| / 7\'7   Xilinx XC9500 I/O Buffer IBIS File
| \ \   Xilinx Inc.
| / /   2100 Logic Drive
| \_\/.\   San Jose,   CA 95124
[IBIS ver]   2.1
[File name]   xc9500.ibs
[File Rev]   1.2
[Date]   June 15, 1999
[Source]   Spice netlist
[Notes]   - max/min process data is not included in this ibis model
   - Control flag setting:
   SLW=0 - fast slew rate
   SLW=1 - slow slew rate
   VIO=0 - 3.3V Vddio
   VIO=1 - 5.0V Vddio
   - Created by Joey Jia x4437
[Disclaimer] The data in this model is derived from SPICE simulations
   using modeling information extracted from the target pro-
   cess. While a great deal of care has been take to provide
   information that is accurate, this model is considered
   preliminary as it has not been verified by actual silicon
   measurement. Treat the data in this model as preliminary
   until actual silicon verification is performed.
[Copyright]   Xilinx Inc.
|   Component XC9536_PLCC44[SLW=0;VIO=0]
[Component]   XC9536_PLCC44[SLW=0;VIO=0]
[Manufacturer]   Xilinx Inc.
[Package]
| variable   typ   min   max
R_pkg   67.500m   66.000m   69.000m
L_pkg   3.910nH   3.550nH   4.260nH
C_pkg   0.895pF   0.790pF   1.000pF
[Pin]  signal_name   model_name   R_pin   L_pin   C_pin
io   iob   IO_00   NA   NA   NA
|   Component XC9536_PLCC44[SLW=1;VIO=0]
[Component]   XC9536_PLCC44[SLW=1;VIO=0]
[Manufacturer]   Xilinx Inc.
[Package]
| variable   typ   min   max
R_pkg   67.500m   66.000m   69.000m
L_pkg   3.910nH   3.550nH   4.260nH
C_pkg   0.895pF   0.790pF   1.000pF
[Pin]  signal_name   model_name   R_pin   L_pin   C_pin
io   iob   IO_10   NA   NA   NA
|   Component XC9536_PLCC44[SLW=0;VIO=1]
[Component]   XC9536_PLCC44[SLW=0;VIO=1]
[Manufacturer]   Xilinx Inc.
[Package]
| variable   typ   min   max
R_pkg   67.500m   66.000m   69.000m
L_pkg   3.910nH   3.550nH   4.260nH
C_pkg   0.895pF   0.790pF   1.000pF
[Pin]  signal_name   model_name   R_pin   L_pin   C_pin
io   iob   IO_01   NA   NA   NA
|   Component XC9536_PLCC44[SLW=1;VIO=1]
[Component]   XC9536_PLCC44[SLW=1;VIO=1]
[Manufacturer]   Xilinx Inc.
[Package]
| variable   typ   min   max
R_pkg   67.500m   66.000m   69.000m
L_pkg   3.910nH   3.550nH   4.260nH
C_pkg   0.895pF   0.790pF   1.000pF
[Pin]  signal_name   model_name   R_pin   L_pin   C_pin
io   iob   IO_11   NA   NA   NA
|   Component XC9536_VQ44[SLW=0;VIO=0]
[Component]   XC9536_VQ44[SLW=0;VIO=0]
[Manufacturer]   Xilinx Inc.
[Package]
| variable   typ   min   max
R_pkg   57.000m   54.000m   60.000m
L_pkg   2.270nH   2.100nH   2.430nH
C_pkg   0.275pF   0.260pF   0.290pF
[Pin]  signal_name   model_name   R_pin   L_pin   C_pin
io   iob   IO_00   NA   NA   NA
| End [Component] XC9536_VQ44[SLW=0;VIO=0]
|   Component XC9536_VQ44[SLW=0;VIO=1]
[Component]   XC9536_VQ44[SLW=0;VIO=1]
[Manufacturer]   Xilinx Inc.
[Package]
| variable   typ   min   max
R_pkg   57.000m   54.000m   60.000m
L_pkg   2.270nH   2.100nH   2.430nH
C_pkg   0.275pF   0.260pF   0.290pF
[Pin]  signal_name   model_name   R_pin   L_pin   C_pin
io   iob   IO_01   NA   NA   NA
| End [Component] XC9536_VQ44[SLW=0;VIO=1]
|   Component XC9536_VQ44[SLW=1;VIO=0]
[Component]   XC9536_VQ44[SLW=1;VIO=0]
[Manufacturer]   Xilinx Inc.
[Package]
| variable   typ   min   max
R_pkg   57.000m   54.000m   60.000m
L_pkg   2.270nH   2.100nH   2.430nH
C_pkg   0.275pF   0.260pF   0.290pF
[Pin]  signal_name   model_name   R_pin   L_pin   C_pin
io   iob   IO_10   NA   NA   NA
| End [Component] XC9536_VQ44[SLW=1;VIO=0]
|   Component XC9536_VQ44[SLW=1;VIO=1]
[Component]   XC9536_VQ44[SLW=1;VIO=1]
[Manufacturer]   Xilinx Inc.
[Package]
| variable   typ   min   max
R_pkg   57.000m   54.000m   60.000m
L_pkg   2.270nH   2.100nH   2.430nH
C_pkg   0.275pF   0.260pF   0.290pF
[Pin]  signal_name   model_name   R_pin   L_pin   C_pin
io   iob   IO_11   NA   NA   NA
| End [Component] XC9536_VQ44[SLW=1;VIO=1]
|   Component XC9572_PLCC44[SLW=0;VIO=0]
[Component]   XC9572_PLCC44[SLW=0;VIO=0]
[Manufacturer]   Xilinx Inc.
[Package]
| variable   typ   min   max
R_pkg   67.500m   66.000m   69.000m
L_pkg   3.910nH   3.550nH   4.260nH
C_pkg   0.895pF   0.790pF   1.000pF
[Pin]  signal_name   model_name   R_pin   L_pin   C_pin
io   iob   IO_00   NA   NA   NA
| End [Component] XC9572_PLCC44[SLW=0;VIO=0]
|   Component XC9572_PLCC44[SLW=0;VIO=1]
[Component]   XC9572_PLCC44[SLW=0;VIO=1]
[Manufacturer]   Xilinx Inc.
[Package]
| variable   typ   min   max
R_pkg   67.500m   66.000m   69.000m
L_pkg   3.910nH   3.550nH   4.260nH
C_pkg   0.895pF   0.790pF   1.000pF
[Pin]  signal_name   model_name   R_pin   L_pin   C_pin
io   iob   IO_01   NA   NA   NA
| End [Component] XC9572_PLCC44[SLW=0;VIO=1]
|   Component XC9572_PLCC44[SLW=1;VIO=0]
[Component]   XC9572_PLCC44[SLW=1;VIO=0]
[Manufacturer]   Xilinx Inc.
[Package]
| variable   typ   min   max
R_pkg   67.500m   66.000m   69.000m
L_pkg   3.910nH   3.550nH   4.260nH
C_pkg   0.895pF   0.790pF   1.000pF
[Pin]  signal_name   model_name   R_pin   L_pin   C_pin
io   iob   IO_10   NA   NA   NA
| End [Component] XC9572_PLCC44[SLW=1;VIO=0]
|   Component XC9572_PLCC44[SLW=1;VIO=1]
[Component]   XC9572_PLCC44[SLW=1;VIO=1]
[Manufacturer]   Xilinx Inc.
[Package]
| variable   typ   min   max
R_pkg   67.500m   66.000m   69.000m
L_pkg   3.910nH   3.550nH   4.260nH
C_pkg   0.895pF   0.790pF   1.000pF
[Pin]  signal_name   model_name   R_pin   L_pin   C_pin
io   iob   IO_11   NA   NA   NA
| End [Component] XC9572_PLCC44[SLW=1;VIO=1]
|   Component XC9572_PLCC84[SLW=0;VIO=0]
[Component]   XC9572_PLCC84[SLW=0;VIO=0]
[Manufacturer]   Xilinx Inc.
[Package]
| variable   typ   min   max
R_pkg   0.104   97.000m   0.111
L_pkg   11.600nH   10.200nH   13.000nH
C_pkg   1.700pF   1.600pF   1.800pF
[Pin]  signal_name   model_name   R_pin   L_pin   C_pin
io   iob   IO_00   NA   NA   NA
| End [Component] XC9572_PLCC84[SLW=0;VIO=0]
|   Component XC9572_PLCC84[SLW=0;VIO=1]
[Component]   XC9572_PLCC84[SLW=0;VIO=1]
[Manufacturer]   Xilinx Inc.
[Package]
| variable   typ   min   max
R_pkg   0.104   97.000m   0.111
L_pkg   11.600nH   10.200nH   13.000nH
C_pkg   1.700pF   1.600pF   1.800pF
[Pin]  signal_name   model_name   R_pin   L_pin   C_pin
io   iob   IO_01   NA   NA   NA
| End [Component] XC9572_PLCC84[SLW=0;VIO=1]
|   Component XC9572_PLCC84[SLW=1;VIO=0]
[Component]   XC9572_PLCC84[SLW=1;VIO=0]
[Manufacturer]   Xilinx Inc.
[Package]
| variable   typ   min   max
R_pkg   0.104   97.000m   0.111
L_pkg   11.600nH   10.200nH   13.000nH
C_pkg   1.700pF   1.600pF   1.800pF
[Pin]  signal_name   model_name   R_pin   L_pin   C_pin
io   iob   IO_10   NA   NA   NA
| End [Component] XC9572_PLCC84[SLW=1;VIO=0]
|   Component XC9572_PLCC84[SLW=1;VIO=1]
[Component]   XC9572_PLCC84[SLW=1;VIO=1]
[Manufacturer]   Xilinx Inc.
[Package]
| variable   typ   min   max
R_pkg   0.104   97.000m   0.111
L_pkg   11.600nH   10.200nH   13.000nH
C_pkg   1.700pF   1.600pF   1.800pF
[Pin]  signal_name   model_name   R_pin   L_pin   C_pin
io   iob   IO_11   NA   NA   NA
| End [Component] XC9572_PLCC84[SLW=1;VIO=1]
|   Component XC9572_PQ100[SLW=0;VIO=0]
[Component]   XC9572_PQ100[SLW=0;VIO=0]
[Manufacturer]   Xilinx Inc.
[Package]
| variable   typ   min   max
R_pkg   88.000m   78.000m   98.000m
L_pkg   6.100nH   4.100nH   8.100nH
C_pkg   0.900pF   0.700pF   1.100pF
[Pin]  signal_name   model_name   R_pin   L_pin   C_pin
io   iob   IO_00   NA   NA   NA
| End [Component] XC9572_PQ100[SLW=0;VIO=0]
|   Component XC9572_PQ100[SLW=0;VIO=1]
[Component]   XC9572_PQ100[SLW=0;VIO=1]
[Manufacturer]   Xilinx Inc.
[Package]
| variable   typ   min   max
R_pkg   88.000m   78.000m   98.000m
L_pkg   6.100nH   4.100nH   8.100nH
C_pkg   0.900pF   0.700pF   1.100pF
[Pin]  signal_name   model_name   R_pin   L_pin   C_pin
io   iob   IO_01   NA   NA   NA
| End [Component] XC9572_PQ100[SLW=0;VIO=1]
|   Component XC9572_PQ100[SLW=1;VIO=0]
[Component]   XC9572_PQ100[SLW=1;VIO=0]
[Manufacturer]   Xilinx Inc.
[Package]
| variable   typ   min   max
R_pkg   88.000m   78.000m   98.000m
L_pkg   6.100nH   4.100nH   8.100nH
C_pkg   0.900pF   0.700pF   1.100pF
[Pin]  signal_name   model_name   R_pin   L_pin   C_pin
io   iob   IO_10   NA   NA   NA
| End [Component] XC9572_PQ100[SLW=1;VIO=0]
|   Component XC9572_PQ100[SLW=1;VIO=1]
[Component]   XC9572_PQ100[SLW=1;VIO=1]
[Manufacturer]   Xilinx Inc.
[Package]
| variable   typ   min   max
R_pkg   88.000m   78.000m   98.000m
L_pkg   6.100nH   4.100nH   8.100nH
C_pkg   0.900pF   0.700pF   1.100pF
[Pin]  signal_name   model_name   R_pin   L_pin   C_pin
io   iob   IO_11   NA   NA   NA
| End [Component] XC9572_PQ100[SLW=1;VIO=1]
|   Component XC9572_TQ100[SLW=0;VIO=0]
[Component]   XC9572_TQ100[SLW=0;VIO=0]
[Manufacturer]   Xilinx Inc.
[Package]
| variable   typ   min   max
R_pkg   84.500m   79.000m   90.000m
L_pkg   4.370nH   3.820nH   4.920nH
C_pkg   0.610pF   0.570pF   0.650pF
[Pin]  signal_name   model_name   R_pin   L_pin   C_pin
io   iob   IO_00   NA   NA   NA
| End [Component] XC9572_TQ100[SLW=0;VIO=0]
|   Component XC9572_TQ100[SLW=0;VIO=1]
[Component]   XC9572_TQ100[SLW=0;VIO=1]
[Manufacturer]   Xilinx Inc.
[Package]
| variable   typ   min   max
R_pkg   84.500m   79.000m   90.000m
L_pkg   4.370nH   3.820nH   4.920nH
C_pkg   0.610pF   0.570pF   0.650pF
[Pin]  signal_name   model_name   R_pin   L_pin   C_pin
io   iob   IO_01   NA   NA   NA
| End [Component] XC9572_TQ100[SLW=0;VIO=1]
|   Component XC9572_TQ100[SLW=1;VIO=0]
[Component]   XC9572_TQ100[SLW=1;VIO=0]
[Manufacturer]   Xilinx Inc.
[Package]
| variable   typ   min   max
R_pkg   84.500m   79.000m   90.000m
L_pkg   4.370nH   3.820nH   4.920nH
C_pkg   0.610pF   0.570pF   0.650pF
[Pin]  signal_name   model_name   R_pin   L_pin   C_pin
io   iob   IO_10   NA   NA   NA
| End [Component] XC9572_TQ100[SLW=1;VIO=0]
|   Component XC9572_TQ100[SLW=1;VIO=1]
[Component]   XC9572_TQ100[SLW=1;VIO=1]
[Manufacturer]   Xilinx Inc.
[Package]
| variable   typ   min   max
R_pkg   84.500m   79.000m   90.000m
L_pkg   4.370nH   3.820nH   4.920nH
C_pkg   0.610pF   0.570pF   0.650pF
[Pin]  signal_name   model_name   R_pin   L_pin   C_pin
io   iob   IO_11   NA   NA   NA
| End [Component] XC9572_TQ100[SLW=1;VIO=1]
|   Component XC95108_PLCC84[SLW=0;VIO=0]
[Component]   XC95108_PLCC84[SLW=0;VIO=0]
[Manufacturer]   Xilinx Inc.
[Package]
| variable   typ   min   max
R_pkg   0.104   97.000m   0.111
L_pkg   11.600nH   10.200nH   13.000nH
C_pkg   1.700pF   1.600pF   1.800pF
[Pin]  signal_name   model_name   R_pin   L_pin   C_pin
io   iob   IO_00   NA   NA   NA
| End [Component] XC95108_PLCC84[SLW=0;VIO=0]
|   Component XC95108_PLCC84[SLW=0;VIO=1]
[Component]   XC95108_PLCC84[SLW=0;VIO=1]
[Manufacturer]   Xilinx Inc.
[Package]
| variable   typ   min   max
R_pkg   0.104   97.000m   0.111
L_pkg   11.600nH   10.200nH   13.000nH
C_pkg   1.700pF   1.600pF   1.800pF
[Pin]  signal_name   model_name   R_pin   L_pin   C_pin
io   iob   IO_01   NA   NA   NA
| End [Component] XC95108_PLCC84[SLW=0;VIO=1]
|   Component XC95108_PLCC84[SLW=1;VIO=0]
[Component]   XC95108_PLCC84[SLW=1;VIO=0]
[Manufacturer]   Xilinx Inc.
[Package]
| variable   typ   min   max
R_pkg   0.104   97.000m   0.111
L_pkg   11.600nH   10.200nH   13.000nH
C_pkg   1.700pF   1.600pF   1.800pF
[Pin]  signal_name   model_name   R_pin   L_pin   C_pin
io   iob   IO_10   NA   NA   NA
| End [Component] XC95108_PLCC84[SLW=1;VIO=0]
|   Component XC95108_PLCC84[SLW=1;VIO=1]
[Component]   XC95108_PLCC84[SLW=1;VIO=1]
[Manufacturer]   Xilinx Inc.
[Package]
| variable   typ   min   max
R_pkg   0.104   97.000m   0.111
L_pkg   11.600nH   10.200nH   13.000nH
C_pkg   1.700pF   1.600pF   1.800pF
[Pin]  signal_name   model_name   R_pin   L_pin   C_pin
io   iob   IO_11   NA   NA   NA
| End [Component] XC95108_PLCC84[SLW=1;VIO=1]
|   Component XC95108_PQ100[SLW=0;VIO=0]
[Component]   XC95108_PQ100[SLW=0;VIO=0]
[Manufacturer]   Xilinx Inc.
[Package]
| variable   typ   min   max
R_pkg   88.000m   78.000m   98.000m
L_pkg   6.100nH   4.100nH   8.100nH
C_pkg   0.900pF   0.700pF   1.100pF
[Pin]  signal_name   model_name   R_pin   L_pin   C_pin
io   iob   IO_00   NA   NA   NA
| End [Component] XC95108_PQ100[SLW=0;VIO=0]
|   Component XC95108_PQ100[SLW=0;VIO=1]
[Component]   XC95108_PQ100[SLW=0;VIO=1]
[Manufacturer]   Xilinx Inc.
[Package]
| variable   typ   min   max
R_pkg   88.000m   78.000m   98.000m
L_pkg   6.100nH   4.100nH   8.100nH
C_pkg   0.900pF   0.700pF   1.100pF
[Pin]  signal_name   model_name   R_pin   L_pin   C_pin
io   iob   IO_01   NA   NA   NA
| End [Component] XC95108_PQ100[SLW=0;VIO=1]
|   Component XC95108_PQ100[SLW=1;VIO=0]
[Component]   XC95108_PQ100[SLW=1;VIO=0]
[Manufacturer]   Xilinx Inc.
[Package]
| variable   typ   min   max
R_pkg   88.000m   78.000m   98.000m
L_pkg   6.100nH   4.100nH   8.100nH
C_pkg   0.900pF   0.700pF   1.100pF
[Pin]  signal_name   model_name   R_pin   L_pin   C_pin
io   iob   IO_10   NA   NA   NA
| End [Component] XC95108_PQ100[SLW=1;VIO=0]
|   Component XC95108_PQ100[SLW=1;VIO=1]
[Component]   XC95108_PQ100[SLW=1;VIO=1]
[Manufacturer]   Xilinx Inc.
[Package]
| variable   typ   min   max
R_pkg   88.000m   78.000m   98.000m
L_pkg   6.100nH   4.100nH   8.100nH
C_pkg   0.900pF   0.700pF   1.100pF
[Pin]  signal_name   model_name   R_pin   L_pin   C_pin
io   iob   IO_11   NA   NA   NA
| End [Component] XC95108_PQ100[SLW=1;VIO=1]
|   Component XC95108_PQ160[SLW=0;VIO=0]
[Component]   XC95108_PQ160[SLW=0;VIO=0]
[Manufacturer]   Xilinx Inc.
[Package]
| variable   typ   min   max
R_pkg   0.194   0.181   0.207
L_pkg   13.300nH   11.300nH   15.200nH
C_pkg   1.700pF   1.500pF   1.900pF
[Pin]  signal_name   model_name   R_pin   L_pin   C_pin
io   iob   IO_00   NA   NA   NA
| End [Component] XC95108_PQ160[SLW=0;VIO=0]
|   Component XC95108_PQ160[SLW=0;VIO=1]
[Component]   XC95108_PQ160[SLW=0;VIO=1]
[Manufacturer]   Xilinx Inc.
[Package]
| variable   typ   min   max
R_pkg   0.194   0.181   0.207
L_pkg   13.300nH   11.300nH   15.200nH
C_pkg   1.700pF   1.500pF   1.900pF
[Pin]  signal_name   model_name   R_pin   L_pin   C_pin
io   iob   IO_01   NA   NA   NA
| End [Component] XC95108_PQ160[SLW=0;VIO=1]
|   Component XC95108_PQ160[SLW=1;VIO=0]
[Component]   XC95108_PQ160[SLW=1;VIO=0]
[Manufacturer]   Xilinx Inc.
[Package]
| variable   typ   min   max
R_pkg   0.194   0.181   0.207
L_pkg   13.300nH   11.300nH   15.200nH
C_pkg   1.700pF   1.500pF   1.900pF
[Pin]  signal_name   model_name   R_pin   L_pin   C_pin
io   iob   IO_10   NA   NA   NA
| End [Component] XC95108_PQ160[SLW=1;VIO=0]
|   Component XC95108_PQ160[SLW=1;VIO=1]
[Component]   XC95108_PQ160[SLW=1;VIO=1]
[Manufacturer]   Xilinx Inc.
[Package]
| variable   typ   min   max
R_pkg   0.194   0.181   0.207
L_pkg   13.300nH   11.300nH   15.200nH
C_pkg   1.700pF   1.500pF   1.900pF
[Pin]  signal_name   model_name   R_pin   L_pin   C_pin
io   iob   IO_11   NA   NA   NA
| End [Component] XC95108_PQ160[SLW=1;VIO=1]
|   Component XC95108_TQ100[SLW=0;VIO=0]
[Component]   XC95108_TQ100[SLW=0;VIO=0]
[Manufacturer]   Xilinx Inc.
[Package]
| variable   typ   min   max
R_pkg   84.500m   79.000m   90.000m
L_pkg   4.370nH   3.820nH   4.920nH
C_pkg   0.610pF   0.570pF   0.650pF
[Pin]  signal_name   model_name   R_pin   L_pin   C_pin
io   iob   IO_00   NA   NA   NA
| End [Component] XC95108_TQ100[SLW=0;VIO=0]
|   Component XC95108_TQ100[SLW=0;VIO=1]
[Component]   XC95108_TQ100[SLW=0;VIO=1]
[Manufacturer]   Xilinx Inc.
[Package]
| variable   typ   min   max
R_pkg   84.500m   79.000m   90.000m
L_pkg   4.370nH   3.820nH   4.920nH
C_pkg   0.610pF   0.570pF   0.650pF
[Pin]  signal_name   model_name   R_pin   L_pin   C_pin
io   iob   IO_01   NA   NA   NA
| End [Component] XC95108_TQ100[SLW=0;VIO=1]
|   Component XC95108_TQ100[SLW=1;VIO=0]
[Component]   XC95108_TQ100[SLW=1;VIO=0]
[Manufacturer]   Xilinx Inc.
[Package]
| variable   typ   min   max
R_pkg   84.500m   79.000m   90.000m
L_pkg   4.370nH   3.820nH   4.920nH
C_pkg   0.610pF   0.570pF   0.650pF
[Pin]  signal_name   model_name   R_pin   L_pin   C_pin
io   iob   IO_10   NA   NA   NA
| End [Component] XC95108_TQ100[SLW=1;VIO=0]
|   Component XC95108_TQ100[SLW=1;VIO=1]
[Component]   XC95108_TQ100[SLW=1;VIO=1]
[Manufacturer]   Xilinx Inc.
[Package]
| variable   typ   min   max
R_pkg   84.500m   79.000m   90.000m
L_pkg   4.370nH   3.820nH   4.920nH
C_pkg   0.610pF   0.570pF   0.650pF
[Pin]  signal_name   model_name   R_pin   L_pin   C_pin
io   iob   IO_11   NA   NA   NA
| End [Component] XC95108_TQ100[SLW=1;VIO=1]
|   Component XC95144_PQ100[SLW=0;VIO=0]
[Component]   XC95144_PQ100[SLW=0;VIO=0]
[Manufacturer]   Xilinx Inc.
[Package]
| variable   typ   min   max
R_pkg   88.000m   78.000m   98.000m
L_pkg   6.100nH   4.100nH   8.100nH
C_pkg   0.900pF   0.700pF   1.100pF
[Pin]  signal_name   model_name   R_pin   L_pin   C_pin
io   iob   IO_00   NA   NA   NA
| End [Component] XC95144_PQ100[SLW=0;VIO=0]
|   Component XC95144_PQ100[SLW=0;VIO=1]
[Component]   XC95144_PQ100[SLW=0;VIO=1]
[Manufacturer]   Xilinx Inc.
[Package]
| variable   typ   min   max
R_pkg   88.000m   78.000m   98.000m
L_pkg   6.100nH   4.100nH   8.100nH
C_pkg   0.900pF   0.700pF   1.100pF
[Pin]  signal_name   model_name   R_pin   L_pin   C_pin
io   iob   IO_01   NA   NA   NA
| End [Component] XC95144_PQ100[SLW=0;VIO=1]
|   Component XC95144_PQ100[SLW=1;VIO=0]
[Component]   XC95144_PQ100[SLW=1;VIO=0]
[Manufacturer]   Xilinx Inc.
[Package]
| variable   typ   min   max
R_pkg   88.000m   78.000m   98.000m
L_pkg   6.100nH   4.100nH   8.100nH
C_pkg   0.900pF   0.700pF   1.100pF
[Pin]  signal_name   model_name   R_pin   L_pin   C_pin
io   iob   IO_10   NA   NA   NA
| End [Component] XC95144_PQ100[SLW=1;VIO=0]
|   Component XC95144_PQ100[SLW=1;VIO=1]
[Component]   XC95144_PQ100[SLW=1;VIO=1]
[Manufacturer]   Xilinx Inc.
[Package]
| variable   typ   min   max
R_pkg   88.000m   78.000m   98.000m
L_pkg   6.100nH   4.100nH   8.100nH
C_pkg   0.900pF   0.700pF   1.100pF
[Pin]  signal_name   model_name   R_pin   L_pin   C_pin
io   iob   IO_11   NA   NA   NA
| End [Component] XC95144_PQ100[SLW=1;VIO=1]
|   Component XC95144_PQ160[SLW=0;VIO=0]
[Component]   XC95144_PQ160[SLW=0;VIO=0]
[Manufacturer]   Xilinx Inc.
[Package]
| variable   typ   min   max
R_pkg   0.194   0.181   0.207
L_pkg   13.300nH   11.300nH   15.200nH
C_pkg   1.700pF   1.500pF   1.900pF
[Pin]  signal_name   model_name   R_pin   L_pin   C_pin
io   iob   IO_00   NA   NA   NA
| End [Component] XC95144_PQ160[SLW=0;VIO=0]
|   Component XC95144_PQ160[SLW=0;VIO=1]
[Component]   XC95144_PQ160[SLW=0;VIO=1]
[Manufacturer]   Xilinx Inc.
[Package]
| variable   typ   min   max
R_pkg   0.194   0.181   0.207
L_pkg   13.300nH   11.300nH   15.200nH
C_pkg   1.700pF   1.500pF   1.900pF
[Pin]  signal_name   model_name   R_pin   L_pin   C_pin
io   iob   IO_01   NA   NA   NA
| End [Component] XC95144_PQ160[SLW=0;VIO=1]
|   Component XC95144_PQ160[SLW=1;VIO=0]
[Component]   XC95144_PQ160[SLW=1;VIO=0]
[Manufacturer]   Xilinx Inc.
[Package]
| variable   typ   min   max
R_pkg   0.194   0.181   0.207
L_pkg   13.300nH   11.300nH   15.200nH
C_pkg   1.700pF   1.500pF   1.900pF
[Pin]  signal_name   model_name   R_pin   L_pin   C_pin
io   iob   IO_10   NA   NA   NA
| End [Component] XC95144_PQ160[SLW=1;VIO=0]
|   Component XC95144_PQ160[SLW=1;VIO=1]
[Component]   XC95144_PQ160[SLW=1;VIO=1]
[Manufacturer]   Xilinx Inc.
[Package]
| variable   typ   min   max
R_pkg   0.194   0.181   0.207
L_pkg   13.300nH   11.300nH   15.200nH
C_pkg   1.700pF   1.500pF   1.900pF
[Pin]  signal_name   model_name   R_pin   L_pin   C_pin
io   iob   IO_11   NA   NA   NA
| End [Component] XC95144_PQ160[SLW=1;VIO=1]
|   Component XC95144_TQ100[SLW=0;VIO=0]
[Component]   XC95144_TQ100[SLW=0;VIO=0]
[Manufacturer]   Xilinx Inc.
[Package]
| variable   typ   min   max
R_pkg   89.500m   84.000m   95.000m
L_pkg   5.200nH   4.700nH   5.700nH
C_pkg   0.650pF   0.600pF   0.700pF
[Pin]  signal_name   model_name   R_pin   L_pin   C_pin
io   iob   IO_00   NA   NA   NA
| End [Component] XC95144_TQ100[SLW=0;VIO=0]
|   Component XC95144_TQ100[SLW=0;VIO=1]
[Component]   XC95144_TQ100[SLW=0;VIO=1]
[Manufacturer]   Xilinx Inc.
[Package]
| variable   typ   min   max
R_pkg   89.500m   84.000m   95.000m
L_pkg   5.200nH   4.700nH   5.700nH
C_pkg   0.650pF   0.600pF   0.700pF
[Pin]  signal_name   model_name   R_pin   L_pin   C_pin
io   iob   IO_01   NA   NA   NA
| End [Component] XC95144_TQ100[SLW=0;VIO=1]
|   Component XC95144_TQ100[SLW=1;VIO=0]
[Component]   XC95144_TQ100[SLW=1;VIO=0]
[Manufacturer]   Xilinx Inc.
[Package]
| variable   typ   min   max
R_pkg   89.500m   84.000m   95.000m
L_pkg   5.200nH   4.700nH   5.700nH
C_pkg   0.650pF   0.600pF   0.700pF
[Pin]  signal_name   model_name   R_pin   L_pin   C_pin
io   iob   IO_10   NA   NA   NA
| End [Component] XC95144_TQ100[SLW=1;VIO=0]
|   Component XC95144_TQ100[SLW=1;VIO=1]
[Component]   XC95144_TQ100[SLW=1;VIO=1]
[Manufacturer]   Xilinx Inc.
[Package]
| variable   typ   min   max
R_pkg   89.500m   84.000m   95.000m
L_pkg   5.200nH   4.700nH   5.700nH
C_pkg   0.650pF   0.600pF   0.700pF
[Pin]  signal_name   model_name   R_pin   L_pin   C_pin
io   iob   IO_11   NA   NA   NA
| End [Component] XC95144_TQ100[SLW=1;VIO=1]
|   Component XC95216_BGA352[SLW=0;VIO=0]
[Component]   XC95216_BGA352[SLW=0;VIO=0]
[Manufacturer]   Xilinx Inc.
[Package]
| variable   typ   min   max
R_pkg   0.225   0.161   0.290
L_pkg   5.500nH   3.800nH   7.200nH
C_pkg   0.950pF   0.700pF   1.200pF
[Pin]  signal_name   model_name   R_pin   L_pin   C_pin
io   iob   IO_00   NA   NA   NA
| End [Component] XC95216_BGA352[SLW=0;VIO=0]
|   Component XC95216_BGA352[SLW=0;VIO=1]
[Component]   XC95216_BGA352[SLW=0;VIO=1]
[Manufacturer]   Xilinx Inc.
[Package]
| variable   typ   min   max
R_pkg   0.225   0.161   0.290
L_pkg   5.500nH   3.800nH   7.200nH
C_pkg   0.950pF   0.700pF   1.200pF
[Pin]  signal_name   model_name   R_pin   L_pin   C_pin
io   iob   IO_01   NA   NA   NA
| End [Component] XC95216_BGA352[SLW=0;VIO=1]
|   Component XC95216_BGA352[SLW=1;VIO=0]
[Component]   XC95216_BGA352[SLW=1;VIO=0]
[Manufacturer]   Xilinx Inc.
[Package]
| variable   typ   min   max
R_pkg   0.225   0.161   0.290
L_pkg   5.500nH   3.800nH   7.200nH
C_pkg   0.950pF   0.700pF   1.200pF
[Pin]  signal_name   model_name   R_pin   L_pin   C_pin
io   iob   IO_10   NA   NA   NA
| End [Component] XC95216_BGA352[SLW=1;VIO=0]
|   Component XC95216_BGA352[SLW=1;VIO=1]
[Component]   XC95216_BGA352[SLW=1;VIO=1]
[Manufacturer]   Xilinx Inc.
[Package]
| variable   typ   min   max
R_pkg   0.225   0.161   0.290
L_pkg   5.500nH   3.800nH   7.200nH
C_pkg   0.950pF   0.700pF   1.200pF
[Pin]  signal_name   model_name   R_pin   L_pin   C_pin
io   iob   IO_11   NA   NA   NA
| End [Component] XC95216_BGA352[SLW=1;VIO=1]
|   Component XC95216_HQ208[SLW=0;VIO=0]
[Component]   XC95216_HQ208[SLW=0;VIO=0]
[Manufacturer]   Xilinx Inc.
[Package]
| variable   typ   min   max
R_pkg   0.146   0.137   0.155
L_pkg   9.450nH   7.110nH   11.790nH
C_pkg   1.930pF   1.780pF   2.070pF
[Pin]  signal_name   model_name   R_pin   L_pin   C_pin
io   iob   IO_00   NA   NA   NA
| End [Component] XC95216_HQ208[SLW=0;VIO=0]
|   Component XC95216_HQ208[SLW=0;VIO=1]
[Component]   XC95216_HQ208[SLW=0;VIO=1]
[Manufacturer]   Xilinx Inc.
[Package]
| variable   typ   min   max
R_pkg   0.146   0.137   0.155
L_pkg   9.450nH   7.110nH   11.790nH
C_pkg   1.930pF   1.780pF   2.070pF
[Pin]  signal_name   model_name   R_pin   L_pin   C_pin
io   iob   IO_01   NA   NA   NA
| End [Component] XC95216_HQ208[SLW=0;VIO=1]
|   Component XC95216_HQ208[SLW=1;VIO=0]
[Component]   XC95216_HQ208[SLW=1;VIO=0]
[Manufacturer]   Xilinx Inc.
[Package]
| variable   typ   min   max
R_pkg   0.146   0.137   0.155
L_pkg   9.450nH   7.110nH   11.790nH
C_pkg   1.930pF   1.780pF   2.070pF
[Pin]  signal_name   model_name   R_pin   L_pin   C_pin
io   iob   IO_10   NA   NA   NA
| End [Component] XC95216_HQ208[SLW=1;VIO=0]
|   Component XC95216_HQ208[SLW=1;VIO=1]
[Component]   XC95216_HQ208[SLW=1;VIO=1]
[Manufacturer]   Xilinx Inc.
[Package]
| variable   typ   min   max
R_pkg   0.146   0.137   0.155
L_pkg   9.450nH   7.110nH   11.790nH
C_pkg   1.930pF   1.780pF   2.070pF
[Pin]  signal_name   model_name   R_pin   L_pin   C_pin
io   iob   IO_11   NA   NA   NA
| End [Component] XC95216_HQ208[SLW=1;VIO=1]
|   Component XC95216_PQ160[SLW=0;VIO=0]
[Component]   XC95216_PQ160[SLW=0;VIO=0]
[Manufacturer]   Xilinx Inc.
[Package]
| variable   typ   min   max
R_pkg   0.172   0.159   0.186
L_pkg   12.450nH   10.700nH   14.200nH
C_pkg   1.450pF   1.300pF   1.600pF
[Pin]  signal_name   model_name   R_pin   L_pin   C_pin
io   iob   IO_00   NA   NA   NA
| End [Component] XC95216_PQ160[SLW=0;VIO=0]
|   Component XC95216_PQ160[SLW=0;VIO=1]
[Component]   XC95216_PQ160[SLW=0;VIO=1]
[Manufacturer]   Xilinx Inc.
[Package]
| variable   typ   min   max
R_pkg   0.172   0.159   0.186
L_pkg   12.450nH   10.700nH   14.200nH
C_pkg   1.450pF   1.300pF   1.600pF
[Pin]  signal_name   model_name   R_pin   L_pin   C_pin
io   iob   IO_01   NA   NA   NA
| End [Component] XC95216_PQ160[SLW=0;VIO=1]
|   Component XC95216_PQ160[SLW=1;VIO=0]
[Component]   XC95216_PQ160[SLW=1;VIO=0]
[Manufacturer]   Xilinx Inc.
[Package]
| variable   typ   min   max
R_pkg   0.172   0.159   0.186
L_pkg   12.450nH   10.700nH   14.200nH
C_pkg   1.450pF   1.300pF   1.600pF
[Pin]  signal_name   model_name   R_pin   L_pin   C_pin
io   iob   IO_10   NA   NA   NA
| End [Component] XC95216_PQ160[SLW=1;VIO=0]
|   Component XC95216_PQ160[SLW=1;VIO=1]
[Component]   XC95216_PQ160[SLW=1;VIO=1]
[Manufacturer]   Xilinx Inc.
[Package]
| variable   typ   min   max
R_pkg   0.172   0.159   0.186
L_pkg   12.450nH   10.700nH   14.200nH
C_pkg   1.450pF   1.300pF   1.600pF
[Pin]  signal_name   model_name   R_pin   L_pin   C_pin
io   iob   IO_11   NA   NA   NA
| End [Component] XC95216_PQ160[SLW=1;VIO=1]
|   Component XC95288_BGA352[SLW=0;VIO=0]
[Component]   XC95288_BGA352[SLW=0;VIO=0]
[Manufacturer]   Xilinx Inc.
[Package]
| variable   typ   min   max
R_pkg   0.225   0.161   0.290
L_pkg   5.500nH   3.800nH   7.200nH
C_pkg   0.950pF   0.700pF   1.200pF
[Pin]  signal_name   model_name   R_pin   L_pin   C_pin
io   iob   IO_00   NA   NA   NA
| End [Component] XC95288_BGA352[SLW=0;VIO=0]
|   Component XC95288_BGA352[SLW=0;VIO=1]
[Component]   XC95288_BGA352[SLW=0;VIO=1]
[Manufacturer]   Xilinx Inc.
[Package]
| variable   typ   min   max
R_pkg   0.225   0.161   0.290
L_pkg   5.500nH   3.800nH   7.200nH
C_pkg   0.950pF   0.700pF   1.200pF
[Pin]  signal_name   model_name   R_pin   L_pin   C_pin
io   iob   IO_01   NA   NA   NA
| End [Component] XC95288_BGA352[SLW=0;VIO=1]
|   Component XC95288_BGA352[SLW=1;VIO=0]
[Component]   XC95288_BGA352[SLW=1;VIO=0]
[Manufacturer]   Xilinx Inc.
[Package]
| variable   typ   min   max
R_pkg   0.225   0.161   0.290
L_pkg   5.500nH   3.800nH   7.200nH
C_pkg   0.950pF   0.700pF   1.200pF
[Pin]  signal_name   model_name   R_pin   L_pin   C_pin
io   iob   IO_10   NA   NA   NA
| End [Component] XC95288_BGA352[SLW=1;VIO=0]
|   Component XC95288_BGA352[SLW=1;VIO=1]
[Component]   XC95288_BGA352[SLW=1;VIO=1]
[Manufacturer]   Xilinx Inc.
[Package]
| variable   typ   min   max
R_pkg   0.225   0.161   0.290
L_pkg   5.500nH   3.800nH   7.200nH
C_pkg   0.950pF   0.700pF   1.200pF
[Pin]  signal_name   model_name   R_pin   L_pin   C_pin
io   iob   IO_11   NA   NA   NA
| End [Component] XC95288_BGA352[SLW=1;VIO=1]
|   Component XC95288_HQ208[SLW=0;VIO=0]
[Component]   XC95288_HQ208[SLW=0;VIO=0]
[Manufacturer]   Xilinx Inc.
[Package]
| variable   typ   min   max
R_pkg   0.106   0.102   0.110
L_pkg   8.900nH   7.900nH   9.900nH
C_pkg   1.650pF   1.500pF   1.800pF
[Pin]  signal_name   model_name   R_pin   L_pin   C_pin
io   iob   IO_00   NA   NA   NA
| End [Component] XC95288_HQ208[SLW=0;VIO=0]
|   Component XC95288_HQ208[SLW=0;VIO=1]
[Component]   XC95288_HQ208[SLW=0;VIO=1]
[Manufacturer]   Xilinx Inc.
[Package]
| variable   typ   min   max
R_pkg   0.106   0.102   0.110
L_pkg   8.900nH   7.900nH   9.900nH
C_pkg   1.650pF   1.500pF   1.800pF
[Pin]  signal_name   model_name   R_pin   L_pin   C_pin
io   iob   IO_01   NA   NA   NA
| End [Component] XC95288_HQ208[SLW=0;VIO=1]
|   Component XC95288_HQ208[SLW=1;VIO=0]
[Component]   XC95288_HQ208[SLW=1;VIO=0]
[Manufacturer]   Xilinx Inc.
[Package]
| variable   typ   min   max
R_pkg   0.106   0.102   0.110
L_pkg   8.900nH   7.900nH   9.900nH
C_pkg   1.650pF   1.500pF   1.800pF
[Pin]  signal_name   model_name   R_pin   L_pin   C_pin
io   iob   IO_10   NA   NA   NA
| End [Component] XC95288_HQ208[SLW=1;VIO=0]
|   Component XC95288_HQ208[SLW=1;VIO=1]
[Component]   XC95288_HQ208[SLW=1;VIO=1]
[Manufacturer]   Xilinx Inc.
[Package]
| variable   typ   min   max
R_pkg   0.106   0.102   0.110
L_pkg   8.900nH   7.900nH   9.900nH
C_pkg   1.650pF   1.500pF   1.800pF
[Pin]  signal_name   model_name   R_pin   L_pin   C_pin
io   iob   IO_11   NA   NA   NA
| End [Component] XC95288_HQ208[SLW=1;VIO=1]
| Models and submodels in the file (4): IO_00 (I/O), IO_10 (I/O), IO_01 (I/O), IO_11 (I/O)
